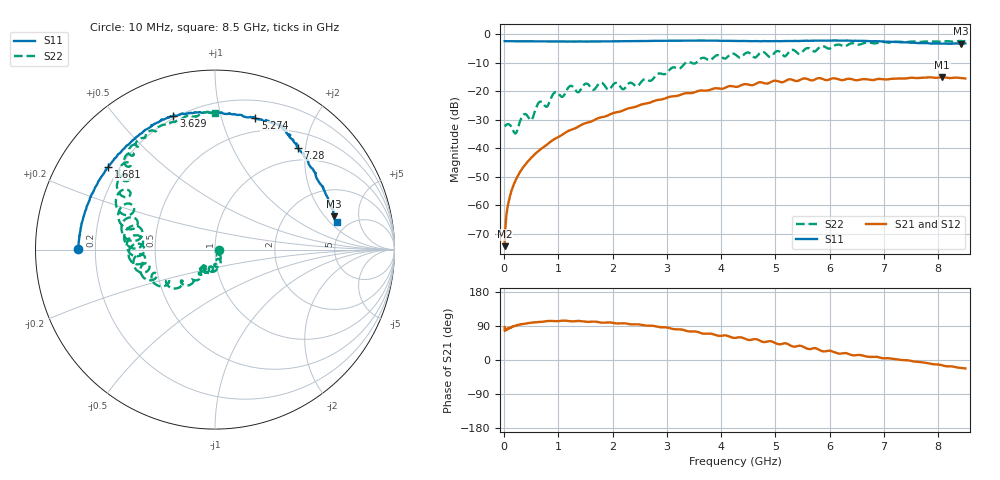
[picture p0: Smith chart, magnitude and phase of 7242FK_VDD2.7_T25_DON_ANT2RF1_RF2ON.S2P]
!Agilent Technologies,E5071C,MY46417908,A.11.23
!Date: Wed Dec 09 15:39:08 2020
!Data & Calibration Information:
!Freq	S11:SOLT2(ON)	S21:SOLT2(ON)	S12:SOLT2(ON)	S22:SOLT2(ON)
!PortZ  Port1:50+j0  Port2:50+j0
!Above PortZ is port z conversion or system Z0 setting when saving the data.
!When reading, reference impedance value at option line is always used.
# Hz S dB R 50
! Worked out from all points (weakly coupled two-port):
!   1601 points, 10 MHz to 8.5 GHz, reference 50 ohm
!   highest |S21| = -14.98 dB at 8.07 GHz (marker M1); lowest = -74.4 dB at 10 MHz (marker M2)
!   lowest |S11| = -3.3 dB at 8.42 GHz (marker M3), VSWR 5.37, Z = 177 + j124 ohm
!   |S11| at or under -10 dB: nowhere
!   |S22| runs from -34.9 to -2.3 dB; largest |S21 - S12| = 0.0021
!   S11 on the Smith chart (normalised r, x): 10 MHz: 0.13, +0.00; 1.681 GHz: 0.16, +0.33; 3.629 GHz: 0.19, +0.72; 5.274 GHz: 0.36, +1.29; 7.28 GHz: 0.76, +1.85; 8.5 GHz: 4.03, +2.43
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1e7  -2.34 179.8  -74.43 86.9  -75.32 81.1  -32.30 -1.6
6.30625e7  -2.37 178.7  -60.91 81.6  -61.18 81.5  -31.52 -18.6
1.16125e8  -2.37 177.5  -56.26 85.0  -56.36 85.7  -31.98 -37.6
2.169438e8  -2.39 175.3  -51.06 90.6  -51.10 91.3  -34.71 -35.1
3.28375e8  -2.40 173.0  -47.27 94.3  -47.35 94.5  -28.99 -40.2
5.034812e8  -2.41 169.3  -43.29 98.4  -43.30 98.5  -30.12 -61.0
6.414438e8  -2.44 166.3  -40.85 100.3  -40.85 100.5  -23.89 -63.3
7.900188e8  -2.46 163.2  -38.72 102.7  -38.71 102.8  -25.37 -72.6
9.385938e8  -2.48 159.8  -36.67 102.7  -36.67 102.7  -20.34 -79.6
1.426769e9  -2.47 148.3  -31.77 102.6  -31.76 102.6  -18.94 -96.2
1.681469e9  -2.47 142.3  -29.86 101.3  -29.87 101.2  -19.00 -107.4
2.450875e9  -2.34 125.7  -25.23 94.2  -25.23 94.3  -18.26 -121.3
2.843538e9  -2.25 118.5  -22.98 87.2  -22.99 87.2  -13.76 -123.3
3.628862e9  -2.16 107.3  -19.67 71.0  -19.68 71.0  -8.41 -148.5
4.255e9  -2.26 96.3  -18.40 58.2  -18.40 58.2  -6.98 -174.7
5.2738e9  -2.32 72.9  -15.78 38.6  -15.75 38.6  -5.69 170.7
5.671769e9  -2.24 65.4  -16.15 29.8  -16.10 29.7  -5.48 151.6
7.088538e9  -2.56 53.9  -15.72 4.6  -15.77 4.4  -2.90 126.6
7.279562e9  -2.72 51.0  -15.47 0.9  -15.46 0.8  -2.55 123.8
8.070194e9  -3.22 26.5  -14.98 -13.7  -15.01 -13.6  -2.50 105.2
8.420406e9  -3.27 15.7  -15.32 -20.9  -15.38 -21.0  -2.33 92.7
8.5e9  -3.15 12.9  -15.49 -22.3  -15.58 -22.1  -2.36 90.1
